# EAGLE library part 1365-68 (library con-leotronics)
DUAL ROW STRAIGHT HEADER 1364 SERIES. 1.27mm x 1.27mm. Without Fixing Post. SMT Source: http://www.leotronics.co.uk/Conexcon/Data%20Sheets/sec.%20A/1364ing.pdf
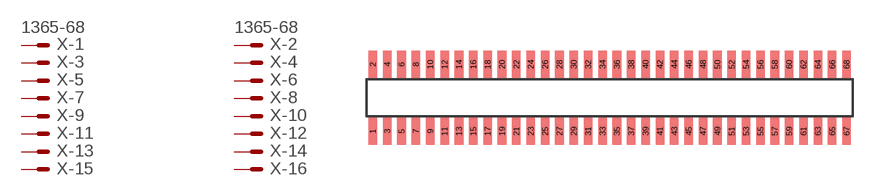
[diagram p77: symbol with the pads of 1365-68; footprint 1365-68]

Designator prefix X; gates -1=MVAL -2=MVAL -3=M -4=M -5=M -6=M -7=M -8=M -9=M -10=M -11=M -12=M -13=M -14=M -15=M -16=M -17=M -18=M -19=M -20=M -21=M -22=M -23=M -24=M -25=M -26=M -27=M -28=M -29=M -30=M -31=M -32=M -33=M -34=M -35=M -36=M -37=M -38=M -39=M -40=M -41=M -42=M -43=M -44=M -45=M -46=M -47=M -48=M -49=M -50=M -51=M -52=M -53=M -54=M -55=M -56=M -57=M -58=M -59=M -60=M -61=M -62=M -63=M -64=M -65=M -66=M -67=M -68=M

## 1365-68 (OC_FARNELL: unknown; OC_NEWARK: unknown)  [1365-68]
1  -1:S  pas
2  -2:S  pas
3  -3:S  pas
4  -4:S  pas
5  -5:S  pas
6  -6:S  pas
7  -7:S  pas
8  -8:S  pas
9  -9:S  pas
10  -10:S  pas
11  -11:S  pas
12  -12:S  pas
13  -13:S  pas
14  -14:S  pas
15  -15:S  pas
16  -16:S  pas
17  -17:S  pas
18  -18:S  pas
19  -19:S  pas
20  -20:S  pas
21  -21:S  pas
22  -22:S  pas
23  -23:S  pas
24  -24:S  pas
25  -25:S  pas
26  -26:S  pas
27  -27:S  pas
28  -28:S  pas
29  -29:S  pas
30  -30:S  pas
31  -31:S  pas
32  -32:S  pas
33  -33:S  pas
34  -34:S  pas
35  -35:S  pas
36  -36:S  pas
37  -37:S  pas
38  -38:S  pas
39  -39:S  pas
40  -40:S  pas
41  -41:S  pas
42  -42:S  pas
43  -43:S  pas
44  -44:S  pas
45  -45:S  pas
46  -46:S  pas
47  -47:S  pas
48  -48:S  pas
49  -49:S  pas
50  -50:S  pas
51  -51:S  pas
52  -52:S  pas
53  -53:S  pas
54  -54:S  pas
55  -55:S  pas
56  -56:S  pas
57  -57:S  pas
58  -58:S  pas
59  -59:S  pas
60  -60:S  pas
61  -61:S  pas
62  -62:S  pas
63  -63:S  pas
64  -64:S  pas
65  -65:S  pas
66  -66:S  pas
67  -67:S  pas
68  -68:S  pas

## Footprint 1365-68 (pad centres in mm)
DUAL ROW STRAIGHT HEADER 1364 SERIES. 1.27mm x 1.27mm. Without Fixing Post. SMT Source: http://www.leotronics.co.uk/Conexcon/Data%20Sheets/sec.%20A/1364ing.pdf
smd 0.76 x 2.4: 1 -20.955,-2.95; 2 -20.955,2.95; 3 -19.685,-2.95; 4 -19.685,2.95; 5 -18.415,-2.95; 6 -18.415,2.95; 7 -17.145,-2.95; 8 -17.145,2.95; 9 -15.875,-2.95; 10 -15.875,2.95; 11 -14.605,-2.95; 12 -14.605,2.95; 13 -13.335,-2.95; 14 -13.335,2.95; 15 -12.065,-2.95; 16 -12.065,2.95; 17 -10.795,-2.95; 18 -10.795,2.95; 19 -9.525,-2.95; 20 -9.525,2.95; 21 -8.255,-2.95; 22 -8.255,2.95; 23 -6.985,-2.95; 24 -6.985,2.95; 25 -5.715,-2.95; 26 -5.715,2.95; 27 -4.445,-2.95; 28 -4.445,2.95; 29 -3.175,-2.95; 30 -3.175,2.95; 31 -1.905,-2.95; 32 -1.905,2.95; 33 -0.635,-2.95; 34 -0.635,2.95; 35 0.635,-2.95; 36 0.635,2.95; 37 1.905,-2.95; 38 1.905,2.95; 39 3.175,-2.95; 40 3.175,2.95; 41 4.445,-2.95; 42 4.445,2.95; 43 5.715,-2.95; 44 5.715,2.95; 45 6.985,-2.95; 46 6.985,2.95; 47 8.255,-2.95; 48 8.255,2.95; 49 9.525,-2.95; 50 9.525,2.95; 51 10.795,-2.95; 52 10.795,2.95; 53 12.065,-2.95; 54 12.065,2.95; 55 13.335,-2.95; 56 13.335,2.95; 57 14.605,-2.95; 58 14.605,2.95; 59 15.875,-2.95; 60 15.875,2.95; 61 17.145,-2.95; 62 17.145,2.95; 63 18.415,-2.95; 64 18.415,2.95; 65 19.685,-2.95; 66 19.685,2.95; 67 20.955,-2.95; 68 20.955,2.95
